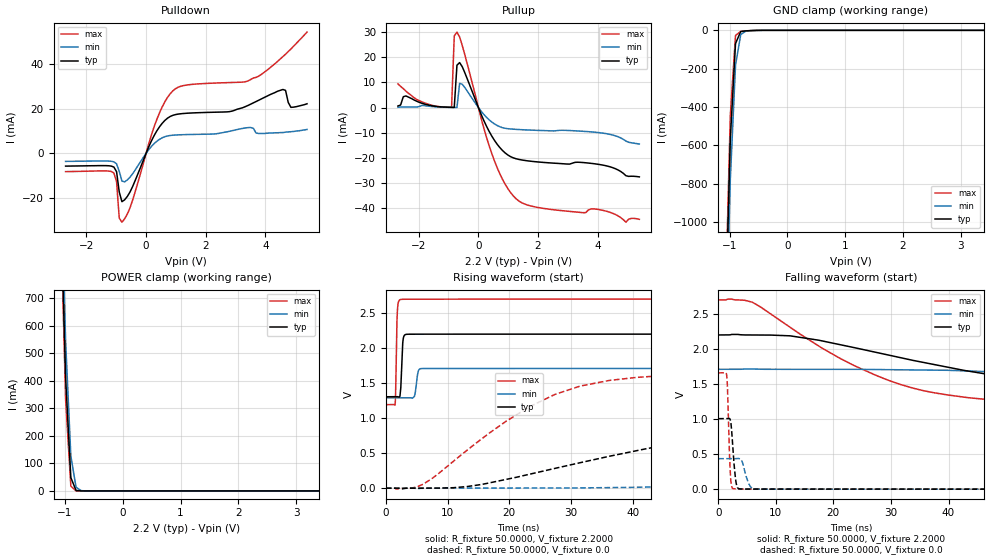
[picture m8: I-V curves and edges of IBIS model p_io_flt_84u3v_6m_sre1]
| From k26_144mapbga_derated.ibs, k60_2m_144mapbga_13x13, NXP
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[Model] p_io_flt_84u3v_6m_sre1
|   Model p_io_flt_84u3v_6m_sre1
| Library cells for typ/min/max conditions are connected as defined below:
|  pad - External Pad
|  ipp_do - Core Input
|  ipp_obe - Output Buffer Enable
|  esd_boost - vdd_s_3v
|  esd_bus - vdd_s_3v
|  ipp_do_3v - vss_bulk
|  ipp_ibe - vss_s_lv
|  ipp_ibe_3v - vss_bulk
|  ipp_ina40a_3v - NC
|  ipp_ina40b_3v - NC
|  ipp_ina_3v - NC
|  ipp_ind - NC
|  ipp_ind_3v - NC
|  ipp_obe1_3v - vss_bulk
|  ipp_pue - vss_s_lv
|  ipp_pue_3v - vss_bulk
|  ipp_pus - vss_s_lv
|  ipp_pus_3v - vss_bulk
|  ipp_sre - vdd_s_lv
|  ipp_sre_3v - vss_bulk
|  ipt_mode_sw_3v - vss_bulk
|  vdd_s_3v - vdd_s_3v
|  vdd_s_lv - vdd_s_lv
|  vss_bulk - vss_bulk
|  vss_s_lv - vss_s_lv
| All other pins connected to ground
Model_type I/O
Polarity   Non-Inverting
Enable   Active-High
Vinl =   0.6600V
Vinh =   1.6500V
Vmeas =  1.1000V
Cref =   25.0000pF
Rref =   50.0000
Vref =   0.0V
C_comp   2.3415pF   2.1611pF   2.5701pF
[Temperature Range]   25.0000   0.1250k   -40.0000
[Voltage Range]   2.2000V   1.7100V   2.7000V
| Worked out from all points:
|   slope of the pulldown table from 0 to 0.33 V, typ, clamps not added: 35.3 ohm
|   slope of the pullup table from 0 to 0.33 V, typ, clamps not added: 37.5 ohm
|   GND clamp passes 1 mA (typ) near -0.60 V on its own axis
|   POWER clamp passes 1 mA (typ) near -0.77 V on its own axis
|   rising waveform, R_fixture 50.0000, V_fixture 2.2000: 20-80 % time 251ps typ, 358ps min, 190ps max; typ from 1.3 V to 2.2 V
|   rising waveform, R_fixture 50.0000, V_fixture 0.0: 20-80 % time 37.3ns typ, 81.2ns min, 16.9ns max; typ from 0 V to 1.01 V
|   falling waveform, R_fixture 50.0000, V_fixture 2.2000: 20-80 % time 37.5ns typ, 76.9ns min, 20.7ns max; typ from 2.2 V to 1.3 V
|   falling waveform, R_fixture 50.0000, V_fixture 0.0: 20-80 % time 571ps typ, 941ps min, 383ps max; typ from 1.01 V to 0 V
[Pulldown]
|Voltage   I(typ)   I(min)   I(max)
-2.7V     -5.71mA    -3.6mA     -8.18mA
-1.08V    -6.144mA   -3.805mA   -8.764mA
-990mV    -8.209mA   -4.705mA   -12.65mA
-900mV    -17.31mA   -8.075mA   -28.99mA
-810mV    -21.63mA   -12.4mA    -30.82mA
-540mV    -17.33mA   -10.67mA   -24.42mA
360mV     10.04mA    5.404mA    15.16mA
900mV     17.03mA    8.127mA    28.01mA
3.69V     23.2mA     9.1mA      34.01mA
4.59V     28.6mA     9.3mA      43.32mA
4.86V     20.6mA     9.7mA      46.7mA
5.4V      22.2mA     10.7mA     54.3mA
[Pullup]
|Voltage   I(typ)   I(min)   I(max)
-2.7V     600uA      100uA      9.4mA
-2.43V    4.6mA      200uA      6.5mA
-900mV    71.6uA     44uA       90.4uA
-810mV    44.44uA    26uA       28.47mA
-720mV    16.81mA    15.9uA     30mA
-630mV    17.86mA    9.617mA    28.04mA
-540mV    16.19mA    9.23mA     24.61mA
450mV     -11.38mA   -5.776mA   -18.35mA
1.17V     -20.01mA   -8.612mA   -35.13mA
1.98V     -21.62mA   -9.083mA   -39.71mA
3.96V     -22.48mA   -9.88mA    -40.43mA
5.4V      -27.58mA   -14.51mA   -44.47mA
[GND_clamp]
|Voltage   I(typ)   I(min)   I(max)
-2.7V     -26.42A    -26.26A    -26.57A
-1.08V    -1.572A    -1.753A    -1.479A
-990mV    -567.4mA   -776.5mA   -443.7mA
-900mV    -68.84mA   -182.9mA   -27.16mA
-810mV    -6.423mA   -22.29mA   -5.195mA
-720mV    -2.652mA   -3.693mA   -3.053mA
-450mV    -86.97uA   -164.9uA   -52.14uA
5.4V      0A         0A         0A
[POWER_clamp]
|Voltage   I(typ)   I(min)   I(max)
-2.7V     17.33A     17.21A     17.45A
-1.08V    1.086A     1.196A     1.032A
-990mV    408mA      540.5mA    329.6mA
-900mV    48.33mA    126.8mA    17.23mA
-810mV    1.793mA    13.06mA    218.7uA
-720mV    55.06uA    999.7uA    2.492uA
-630mV    1.661uA    73.44uA    28.49nA
5.4V      0A         0A         0A
[Ramp]
| variable   typ   min   max
dV/dt_r  0.6035/37.3069n   0.2592/81.1358n   0.9955/16.9144n
dV/dt_f  0.5371/37.4649n   0.2505/76.8648n   0.9044/20.7424n
R_load = 50.0000
[Rising Waveform]
R_fixture= 50.0000
V_fixture= 2.2000
V_fixture_min= 1.7100
V_fixture_max= 2.7000
|time   V(typ)   V(min)   V(max)
0s        1.305V     1.291V     1.193V
1.495ns   1.305V     1.291V     1.196V
1.885ns   1.306V     1.291V     2.553V
2.283ns   1.313V     1.291V     2.69V
2.611ns   1.863V     1.291V     2.697V
3.015ns   2.183V     1.291V     2.698V
4.624ns   2.199V     1.309V     2.698V
5.266ns   2.199V     1.674V     2.698V
6.306ns   2.199V     1.709V     2.698V
300ns     2.2V       1.71V      2.7V
[Rising Waveform]
R_fixture= 50.0000
V_fixture= 0.0
V_fixture_min= 0.0
V_fixture_max= 0.0
|time   V(typ)   V(min)   V(max)
0s        1.247nV    38.99nV    73.88pV
6.04ns    -107.4uV   -1.019mV   56.99mV
19.47ns   123.9mV    46.54uV    954.8mV
27.38ns   282.1mV    1.02mV     1.338V
36.26ns   456.4mV    7.44mV     1.539V
45.8ns    618mV      23.22mV    1.611V
63.88ns   838.7mV    82.97mV    1.648V
91.52ns   964.4mV    190.4mV    1.658V
176.1ns   1.005V     387.8mV    1.659V
300ns     1.006V     432mV      1.659V
[Falling Waveform]
R_fixture= 50.0000
V_fixture= 2.2000
V_fixture_min= 1.7100
V_fixture_max= 2.7000
|time   V(typ)   V(min)   V(max)
0s        2.2V       1.71V      2.7V
5.932ns   2.2V       1.714V     2.667V
18.01ns   2.116V     1.71V      2.014V
29.42ns   1.916V     1.706V     1.557V
37.63ns   1.776V     1.699V     1.373V
48.8ns    1.613V     1.671V     1.264V
77.39ns   1.38V      1.569V     1.198V
107.4ns   1.321V     1.458V     1.192V
174.2ns   1.306V     1.328V     1.193V
300ns     1.305V     1.292V     1.193V
[Falling Waveform]
R_fixture= 50.0000
V_fixture= 0.0
V_fixture_min= 0.0
V_fixture_max= 0.0
|time   V(typ)   V(min)   V(max)
0s        1.006V     434.9mV    1.659V
1.489ns   1.006V     434.7mV    1.619V
1.609ns   1.006V     434.6mV    1.454V
1.995ns   1.005V     434.5mV    426.2mV
2.188ns   950.5mV    434.4mV    126.8mV
3.047ns   127.4mV    435.3mV    3.787mV
4.04ns    2.144mV    414.3mV    1.977mV
5.558ns   1.06mV     40.29mV    1.919mV
6.911ns   1.031mV    1.419mV    1.576mV
300ns     1.375uV    785.7nV    1.114uV
